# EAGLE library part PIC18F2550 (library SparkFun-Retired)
PIC18F2550 Retired: IC-08240
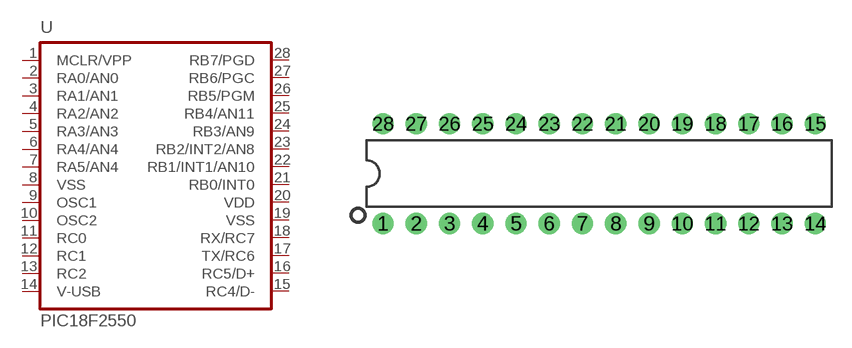
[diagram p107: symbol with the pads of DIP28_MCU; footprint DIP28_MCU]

Designator prefix -

## PIC18F2550  [DIP28_MCU]
1  MCLR/VPP
2  RA0/AN0
3  RA1/AN1
4  RA2/AN2
5  RA3/AN3
6  RA4/AN4
7  RA5/AN4
8  VSS  pwr
9  OSC1
10  OSC2
11  RC0
12  RC1
13  RC2
14  V-USB
15  RC4/D-
16  RC5/D+
17  TX/RC6
18  RX/RC7  in
19  VSS  pwr
20  VDD  pwr
21  RB0/INT0
22  RB1/INT1/AN10
23  RB2/INT2/AN8
24  RB3/AN9
25  RB4/AN11
26  RB5/PGM
27  RB6/PGC
28  RB7/PGD

## Footprint DIP28_MCU (pad centres in mm)
Standard 28-pin DIP package. IC needs to have legs bent before insertion.
drill 0.813 pad 1.626: 1 -16.51,-3.81; 2 -13.97,-3.81; 3 -11.43,-3.81; 4 -8.89,-3.81; 5 -6.35,-3.81; 6 -3.81,-3.81; 7 -1.27,-3.81; 8 1.27,-3.81; 9 3.81,-3.81; 10 6.35,-3.81; 11 8.89,-3.81; 12 11.43,-3.81; 13 13.97,-3.81; 14 16.51,-3.81; 15 16.51,3.81; 16 13.97,3.81; 17 11.43,3.81; 18 8.89,3.81; 19 6.35,3.81; 20 3.81,3.81; 21 1.27,3.81; 22 -1.27,3.81; 23 -3.81,3.81; 24 -6.35,3.81; 25 -8.89,3.81; 26 -11.43,3.81; 27 -13.97,3.81; 28 -16.51,3.81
